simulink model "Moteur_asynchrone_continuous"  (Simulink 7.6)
settings: Solver=ode15s  StartTime=0.0  StopTime=150  MaxStep=1/60  RelTol=1e-4  AbsTol=1e-4
InitFcn:
  | clear all
  | close all
  | clc
StopFcn:
  | close all
  | load Istator_Vitesse.mat
  | 
  | plotyy(x(1,:),x(2,:), x(1,:),x(3,:))
  | title('Courant statorique et vitesse de rotation')
  | grid
  | xlabel('temps')
libraries: powerlib x5

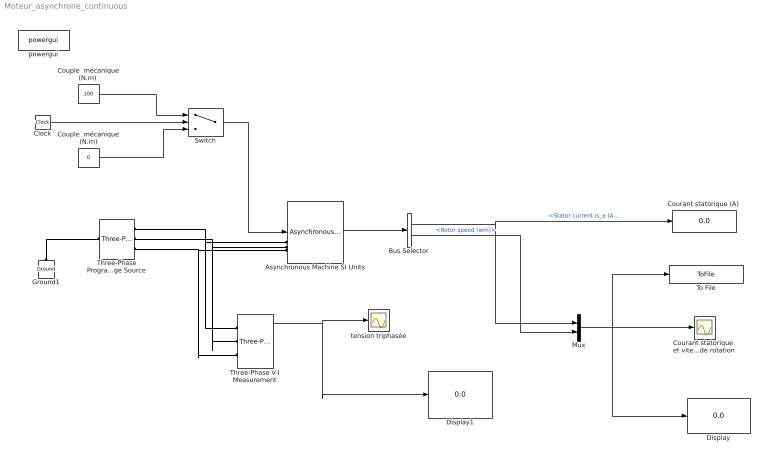
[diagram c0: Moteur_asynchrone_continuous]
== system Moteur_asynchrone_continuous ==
  Asynchronous Machine SI Units : powerlib/Machines/Asynchronous Machine SI Units  DialogController=POWERSYS.PowerSysDialog  SystemSampleTime=-1  PresetModel=No  MechanicalLoad=Torque Tm  ShowDetailedParameters=on  RotorType=Squirrel-cage  ReferenceFrame=Rotor  NominalParameters=[ 3800, 380, 60 ]  Stator=[ 0.029 0.226/377]  Rotor=[ 0.022 0.226/377]  Cage1=[ 0.022 0.226/377]  Cage2=[ 0.022 0.226/377]  Lm=13.04/377  Mechanical="[ 63.87 0  2 ]"  PolePairs=2  InitialConditions=[1 0 0 0 0 0 0 0]  Units=SI  LoadFlowParameters=1492000  SimulateSaturation=off  Saturation=[14.03593122, 27.81365428, 53.79336849, 72.68890987, 97.98006896, 148.6815601, 215.7428561, 302.9841135, 428.7778367 ; 230, 322, 414, 460, 506, 552, 598, 644, 690]  TsPowergui=0  TsBlock=-1  IterativeModel=Forward Euler
  Bus Selector : BusSelector  OutputSignals=Stator measurements.Stator current is_a (A),Mechanical.Rotor speed (wm)
  Clock : Clock
  Couple  mécanique (N.m) : Constant  Value=0
  "Couple  mécanique (N.m) " : Constant  Value=100
  "Courant statorique (A) " : Display
  Courant statorique  et vitesse de rotation : Scope
  Display : Display
  Display1 : Display
  Ground1 : powerlib/Elements/Ground  DialogController=POWERSYS.PowerSysDialog  PhysicalDomain=powersysdomain  SubClassName=unknown  LeftPortType=p1  RightPortType=p1  LConnTagsString=a
  Mux : Mux  Inputs=2
  Switch : Switch  Threshold=50
  Three-Phase V-I Measurement : powerlib/Measurements/Three-Phase V-I Measurement  DialogController=POWERSYS.PowerSysDialog  SystemSampleTime=-1  VoltageMeasurement=phase-to-ground  SetLabelV=off  LabelV=Vabc  Vpu=off  VpuLL=off  CurrentMeasurement=yes  SetLabelI=off  LabelI=Iabc  Ipu=off  Pbase=100e6  Vbase=500e3  OutputType=Magnitude  PhasorSimulation=off  PSBequivalent=0
  Three-Phase Programmable  Voltage Source : powerlib/Electrical Sources/Three-Phase Programmable Voltage Source  DialogController=POWERSYS.PowerSysDialog  SystemSampleTime=-1  PositiveSequence="[380  0 60]"  VariationEntity=Amplitude  VariationType=Step  VariationStep=0.5  VariationRate=10  VariationMagnitude=0.3  VariationFrequency=2  VariationTiming=[10 30]  VariationPhaseA=off  Amplitudes=[1 0.8 1.2 1.0]  TimeValues=[0 0.1 0.15 0.2]  HarmonicGeneration=off  HarmonicA=[3 0.2 -25 0]  HarmonicB=[2 0.15 35 2]  Timing="[0.05  3]"
  To File : ToFile  Filename=Istator_Vitesse  MatrixName=x
  powergui : powerlib/powergui  Priority=2  SystemSampleTime=-1  SimulationMode=Continuous  SampleTime=1e-5  frequency=60  SPID=off  DisableSnubberDevices=off  DisableRonSwitches=off  DisableVfSwitches=off  SwTol=0  Interpol=off  frequencyindice=60  echomessages=off  HookPort=off  DisplayEquations=off  FunctionMessages=off  EnableUseOfTLC=off  x0status=blocks  RestoreLinks=warning  ResistiveCurrentMeasurement=off  Frange=[0:2:500]  Ylog=off  Xlog=on  ShowGrid=off  save=off  variable=ZData  ZoomFFT=on  StartTime=0.0  cycles=1  DisplayStyle=1  fundamental=60  FreqAxis=off  MaxFrequency=1000  frequencyindicesteady=1  RmsSteady=1  display=off  Ts=0  methode=off
  tension triphasée : Scope
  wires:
  Asynchronous Machine SI Units/1 -> Bus Selector/1
  Mux/1 -> Courant statorique  et vitesse de rotation/1, To File/1, Display/1
  Bus Selector/1 -> Mux/1, "Courant statorique (A) "/1  "<Stator current is_a (A)>"
  Bus Selector/2 -> Mux/2  "<Rotor speed (wm)>"
  Three-Phase V-I Measurement/1 -> tension triphasée/1, Display1/1
  Couple  mécanique (N.m)/1 -> Switch/3
  Clock/1 -> Switch/2
  "Couple  mécanique (N.m) "/1 -> Switch/1
  Switch/1 -> Asynchronous Machine SI Units/1
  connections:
  Three-Phase Programmable  Voltage Source/RConn1 -- Asynchronous Machine SI Units/LConn1 -- Three-Phase V-I Measurement/LConn1
  Asynchronous Machine SI Units/LConn2 -- Three-Phase Programmable  Voltage Source/RConn2 -- Three-Phase V-I Measurement/LConn2
  Asynchronous Machine SI Units/LConn3 -- Three-Phase Programmable  Voltage Source/RConn3 -- Three-Phase V-I Measurement/LConn3
  Ground1/LConn1 -- Three-Phase Programmable  Voltage Source/LConn1
